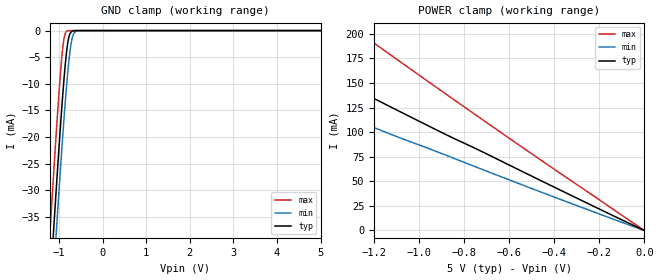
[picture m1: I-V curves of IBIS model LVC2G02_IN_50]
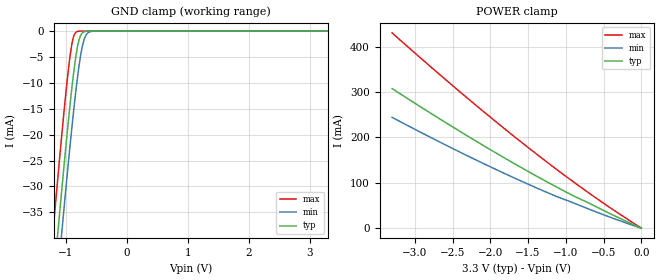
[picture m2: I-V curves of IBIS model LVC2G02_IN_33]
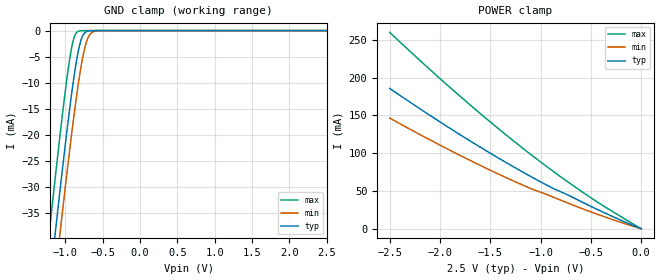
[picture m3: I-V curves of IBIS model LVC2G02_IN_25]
| TEXAS INSTRUMENTS INCORPORATED
| Standard Linear and Logic Group
| IBIS Model of SN74LVC2G02
| DUAL 2-INPUT POSITIVE-NOR GATE
| This file contains package information for the following:
|  SSOP 8-pin (DCT) package as [Component] LVC2G02_DCT
|  VSSOP 8-pin (DCU) package as [Component] LVC2G02_DCU
|  NanoStar WCSP 8-pin (YEA) package as [Component] LVC2G02_YEA
|  NanoFree WCSP 8-pin (YZA) package as [Component] LVC2G02_YZA
|  NanoStar WCSP 8-pin (YEP) package as [Component] LVC2G02_YEP
|  NanoFree WCSP 8-pin (YZP) package as [Component] LVC2G02_YZP
| This device can be powered at the following Vccs:
|  5 volt Vcc
|  3.3 volt Vcc
|  2.5 volt Vcc
|  1.8 volt Vcc
| This file provides unique models under the [Model Selector] for each Vcc.
| For operation at a specific Vcc, select the appropriate model after each
| [Model Selector] keyword.
[IBIS Ver]   3.2
[Comment char]  |_char
[File Name]   sn74lvc2g02.ibs
[File Rev]   1.2 | d_die
[Date]   August 18, 2003
[Source]   Data created from TI-SPICE simulations at TI-SLL.
[Notes]   The following is an IBIS list for the LVC2G02.
   Please contact sllibis@ti.com with questions and
   comments concerning SLL IBIS models.
[Disclaimer] Property of Texas Instruments Incorporated.  Unauthorized
   reproduction and/or distribution is strictly prohibited.
   This product is protected under copyright law.
   Created  2002, (C) Copyright  2002, Texas Instruments
   Incorporated, All Rights Reserved
   UNLESS THERE IS A SIGNED, WRITTEN AGREEMENT TO THE
   CONTRARY, TEXAS INSTRUMENTS (TI) IS PROVIDING THE IBIS
   MODELS  AND WITHOUT ANY WARRANTY, EXPRESSED OR
   IMPLIED.  TI assumes no liability for:
   1) the accuracy of the IBIS models provided to your
   company;
   2) the proper functioning of these IBIS Models in your
   design or for any resulting applications; or
   3) infringement of patents, copyrights or intellectual
   property rights resulting from your use of these IBIS
   models.
   TI provides IBIS Models as a service to our customers.
   You and your company shall not distribute, sell or give
   these models to anyone else without prior written
   permission from TI.
   TI reserves the right to make changes to our products or
   to discontinue any semiconductor product or service
   without notice, and advises our customers to obtain the
   latest version of relevant information to verify, before
   placing orders, that the information being relied on is
   current.
   Please be aware that your receipt and use of the IBIS
   information provided shall serve as acceptance of these
   terms and conditions.  If you do not accept these terms,
   you should return or destroy the IBIS models and any
   other accompanying information immediately.
| Component LVC2G02_DCT 8-pin TSSOP
[Component]   LVC2G02_DCT
[Manufacturer]   Texas Instruments, Inc.
[Package]
|   typ   min   max
R_pkg   2.900e-02   2.800e-02   3.100e-02
L_pkg   1.796e-09   1.666e-09   1.924e-09
C_pkg   1.090e-13   8.300e-14   1.360e-13
[Pin]   signal_name   model_name   R_pin   L_pin   C_pin
1   1A   LVC2G02_IN   3.100e-02   1.894e-09   1.340e-13
2   1B   LVC2G02_IN   2.800e-02   1.697e-09   8.600e-14
3   2Y   LVC2G02_OUT   3.000e-02   1.722e-09   8.600e-14
4   GND   GND   3.000e-02   1.861e-09   1.300e-13
5   2A   LVC2G02_IN   2.800e-02   1.924e-09   1.360e-13
6   2B   LVC2G02_IN   2.900e-02   1.736e-09   8.600e-14
7   1Y   LVC2G02_OUT   2.800e-02   1.666e-09   8.300e-14
8   VCC   POWER   3.000e-02   1.871e-09   1.320e-13
| Component LVC2G02_DCU 8-pin SOT
[Component]   LVC2G02_DCU
[Manufacturer]   Texas Instruments, Inc.
[Package]
|   typ   min   max
R_pkg   2.600e-02   2.300e-02   3.800e-02
L_pkg   1.394e-09   1.066e-09   2.046e-09
C_pkg   2.590e-13   2.150e-13   3.720e-13
[Pin]   signal_name   model_name   R_pin   L_pin   C_pin
1   1A   LVC2G02_IN   2.400e-02   1.520e-09   2.710e-13
2   1B   LVC2G02_IN   2.300e-02   1.112e-09   2.180e-13
3   2Y   LVC2G02_OUT   2.300e-02   1.070e-09   2.170e-13
4   GND   GND   2.700e-02   2.046e-09   3.720e-13
5   2A   LVC2G02_IN   2.700e-02   1.542e-09   2.730e-13
6   2B   LVC2G02_IN   2.300e-02   1.100e-09   2.240e-13
7   1Y   LVC2G02_OUT   2.300e-02   1.066e-09   2.150e-13
8   VCC   POWER   3.800e-02   1.696e-09   2.800e-13
| Component LVC2G02_YEA 8-pin NanoStar WCSP
[Component]   LVC2G02_YEA
[Manufacturer]   Texas Instruments, Inc.
[Package]
|   typ   min   max
R_pkg   0.001   0.001   0.001
L_pkg   0.021nH   0.021nH   0.021nH
C_pkg   0.043pF   0.042pF   0.044pF
[Pin]   signal_name   model_name   R_pin   L_pin   C_pin
1   1A   LVC2G02_IN   0.046   2.861nH   0.321pF
2   1B   LVC2G02_IN   0.037   2.437nH   0.286pF
3   2Y   LVC2G02_OUT   0.034   2.419nH   0.286pF
4   GND   GND   0.043   2.784nH   0.321pF
5   2A   LVC2G02_IN   0.043   2.784nH   0.321pF
6   2B   LVC2G02_IN   0.035   2.420nH   0.286pF
7   1Y   LVC2G02_OUT   0.037   2.437nH   0.286pF
8   VCC   POWER   0.046   2.860nH   0.321pF
| Component LVC2G02_YZA 8-pin NanoFree WCSP
[Component]   LVC2G02_YZA
[Manufacturer]   Texas Instruments, Inc.
[Package]
|   typ   min   max
R_pkg   0.001   0.001   0.001
L_pkg   0.021nH   0.021nH   0.021nH
C_pkg   0.043pF   0.042pF   0.044pF
[Pin]   signal_name   model_name   R_pin   L_pin   C_pin
1   1A   LVC2G02_IN   0.046   2.861nH   0.321pF
2   1B   LVC2G02_IN   0.037   2.437nH   0.286pF
3   2Y   LVC2G02_OUT   0.034   2.419nH   0.286pF
4   GND   GND   0.043   2.784nH   0.321pF
5   2A   LVC2G02_IN   0.043   2.784nH   0.321pF
6   2B   LVC2G02_IN   0.035   2.420nH   0.286pF
7   1Y   LVC2G02_OUT   0.037   2.437nH   0.286pF
8   VCC   POWER   0.046   2.860nH   0.321pF
| Component LVC2G02_YEP 8-pin NanoStar WCSP
[Component]   LVC2G02_YEP
[Manufacturer]   Texas Instruments, Inc.
[Package]
|   typ   min   max
R_pkg   0.001   0.001   0.001
L_pkg   0.021nH   0.021nH   0.021nH
C_pkg   0.043pF   0.042pF   0.044pF
[Pin]   signal_name   model_name   R_pin   L_pin   C_pin
1   1A   LVC2G02_IN   0.046   2.861nH   0.321pF
2   1B   LVC2G02_IN   0.037   2.437nH   0.286pF
3   2Y   LVC2G02_OUT   0.034   2.419nH   0.286pF
4   GND   GND   0.043   2.784nH   0.321pF
5   2A   LVC2G02_IN   0.043   2.784nH   0.321pF
6   2B   LVC2G02_IN   0.035   2.420nH   0.286pF
7   1Y   LVC2G02_OUT   0.037   2.437nH   0.286pF
8   VCC   POWER   0.046   2.860nH   0.321pF
| Component LVC2G02_YZP 8-pin NanoFree WCSP
[Component]   LVC2G02_YZP
[Manufacturer]   Texas Instruments, Inc.
[Package]
|   typ   min   max
R_pkg   0.001   0.001   0.001
L_pkg   0.021nH   0.021nH   0.021nH
C_pkg   0.043pF   0.042pF   0.044pF
[Pin]   signal_name   model_name   R_pin   L_pin   C_pin
1   1A   LVC2G02_IN   0.046   2.861nH   0.321pF
2   1B   LVC2G02_IN   0.037   2.437nH   0.286pF
3   2Y   LVC2G02_OUT   0.034   2.419nH   0.286pF
4   GND   GND   0.043   2.784nH   0.321pF
5   2A   LVC2G02_IN   0.043   2.784nH   0.321pF
6   2B   LVC2G02_IN   0.035   2.420nH   0.286pF
7   1Y   LVC2G02_OUT   0.037   2.437nH   0.286pF
8   VCC   POWER   0.046   2.860nH   0.321pF
| Model LVC2G02_IN
[Model Selector]   LVC2G02_IN
LVC2G02_IN_50   5 volt Vcc
LVC2G02_IN_33   3.3 volt Vcc
LVC2G02_IN_25   2.5 volt Vcc
LVC2G02_IN_18   1.8 volt Vcc
| Model LVC2G02_OUT
[Model Selector]   LVC2G02_OUT
LVC2G02_OUT_50   5 volt Vcc
LVC2G02_OUT_33   3.3 volt Vcc
LVC2G02_OUT_25   2.5 volt Vcc
LVC2G02_OUT_18   1.8 volt Vcc
| Models and submodels in the file (8): LVC2G02_IN_50 (Input), LVC2G02_IN_33 (Input), LVC2G02_IN_25 (Input), LVC2G02_IN_18 (Input), LVC2G02_OUT_50 (Output), LVC2G02_OUT_33 (Output), LVC2G02_OUT_25 (Output), LVC2G02_OUT_18 (Output)
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[Model]   LVC2G02_IN_50
Model_type  Input
Vinl=1.35
Vinh=3.85
| variable   typ   min   max
C_comp   5.00pF   NA   NA
[Temperature Range]   40   100   -40
| Ambient temperature   25   85   -40
[Voltage range]   5   4.5   5.5
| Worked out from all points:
|   GND clamp passes 1 mA (typ) near -0.77 V on its own axis
|   POWER clamp passes 1 mA (typ) near -0.01 V on its own axis
[GND Clamp]
| LVC2G02_IN_50
|   Voltage   I(typ)   I(min)   I(max)
-5.5V     -655.2mA   -662.2mA   -646.6mA
-1.215V   -49.6mA    -57.88mA   -38.96mA
-1.135V   -39.07mA   -47.36mA   -28.42mA
-1.115V   -36.48mA   -44.76mA   -25.84mA
-1.055V   -28.82mA   -37.05mA   -18.27mA
-915mV    -12.21mA   -19.95mA   -3.333mA
-870mV    -7.651mA   -14.9mA    -891.1uA
-815mV    -3.252mA   -9.299mA   -87.06uA
-770mV    -1.128mA   -5.445mA   -10.73uA
-705mV    -146.7uA   -1.723mA   -505nA
-575mV    -1.597uA   -52.97uA   -1.117nA
5V        9.69pA     12.83pA    9.218pA
[POWER Clamp]
| LVC2G02_IN_50
|   Voltage   I(typ)   I(min)   I(max)
-5V       610.5mA    490.7mA    849.3mA
-2.285V   264.1mA    208.3mA    372.2mA
-2.205V   254.3mA    200.4mA    358.5mA
-1.825V   208.2mA    163.5mA    294.2mA
-1.75V    199.2mA    156.3mA    281.7mA
-1.295V   145.2mA    113.4mA    206.1mA
-1.255V   140.6mA    109.7mA    199.5mA
-905mV    100.2mA    78.68mA    142.6mA
-640mV    71.05mA    54.98mA    100.1mA
-84.45fV  14.56pA    244.4pA    504.6pA
[Model]   LVC2G02_IN_33
Model_type  Input
Vinl=0.8
Vinh=2.0
| variable   typ   min   max
C_comp   5.00pF   NA   NA
[Temperature Range]   40   100   -40
| Ambient temperature   25   85   -40
[Voltage range]   3.3   3   3.6
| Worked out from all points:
|   GND clamp passes 1 mA (typ) near -0.77 V on its own axis
|   POWER clamp passes 1 mA (typ) near -0.01 V on its own axis
[GND Clamp]
| LVC2G02_IN_33
|   Voltage   I(typ)   I(min)   I(max)
-5.5V     -655.2mA   -662.2mA   -646.6mA
-1.225V   -50.93mA   -59.21mA   -40.3mA
-1.145V   -40.37mA   -48.66mA   -29.72mA
-1.12V    -37.12mA   -45.41mA   -26.48mA
-1.08V    -31.98mA   -40.25mA   -21.38mA
-1.06V    -29.44mA   -37.69mA   -18.89mA
-965mV    -17.84mA   -25.87mA   -7.89mA
-885mV    -9.098mA   -16.55mA   -1.486mA
-780mV    -1.472mA   -6.227mA   -17.15uA
-715mV    -205.4uA   -2.128mA   -808.5nA
-640mV    -15.53uA   -338.1uA   -23.69nA
3.3V      6.304pA    9.258pA    5.93pA
[POWER Clamp]
| LVC2G02_IN_33
|   Voltage   I(typ)   I(min)   I(max)
-3.3V     307.9mA    244.4mA    430.7mA
-2.345V   207.8mA    163.1mA    292.8mA
-1.485V   123.9mA    95.99mA    176.1mA
-990mV    79.2mA     61.62mA    113.3mA
-715mV    56.95mA    43.47mA    80.08mA
-48.03fV  10.78pA    241.1pA    451pA
[Model]   LVC2G02_IN_25
Model_type  Input
Vinl=0.7
Vinh=1.7
| variable   typ   min   max
C_comp   5.00pF   NA   NA
[Temperature Range]   40   100   -40
| Ambient temperature   25   85   -40
[Voltage range]   2.5   2.3   2.7
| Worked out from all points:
|   GND clamp passes 1 mA (typ) near -0.77 V on its own axis
|   POWER clamp passes 1 mA (typ) near -0.02 V on its own axis
[GND Clamp]
| LVC2G02_IN_25
|   Voltage   I(typ)   I(min)   I(max)
-5.5V     -655.2mA   -662.2mA   -646.6mA
-1.215V   -49.6mA    -57.88mA   -38.96mA
-1.14V    -39.72mA   -48.01mA   -29.07mA
-1.12V    -37.12mA   -45.41mA   -26.48mA
-1.08V    -31.98mA   -40.25mA   -21.38mA
-1.06V    -29.44mA   -37.69mA   -18.89mA
-960mV    -17.26mA   -25.26mA   -7.377mA
-890mV    -9.597mA   -17.1mA    -1.734mA
-785mV    -1.671mA   -6.635mA   -21.67uA
-720mV    -242.5uA   -2.354mA   -1.023uA
-650mV    -22.01uA   -443.9uA   -37.93nA
2.5V      4.713pA    7.577pA    4.389pA
[POWER Clamp]
| LVC2G02_IN_25
|   Voltage   I(typ)   I(min)   I(max)
-2.5V     185.9mA    146.6mA    260.1mA
-2.14V    153.6mA    120.5mA    215.7mA
-1.775V   122.4mA    95.36mA    172.5mA
-1.465V   97.17mA    75.24mA    137.5mA
-1.15V    72.98mA    56.11mA    103.8mA
-890mV    54.36mA    42.66mA    77.46mA
-560mV    33.45mA    25.2mA     46.32mA
-330mV    18.9mA     14.11mA    26.4mA
-31.15fV  8.992pA    239.5pA    424.3pA
